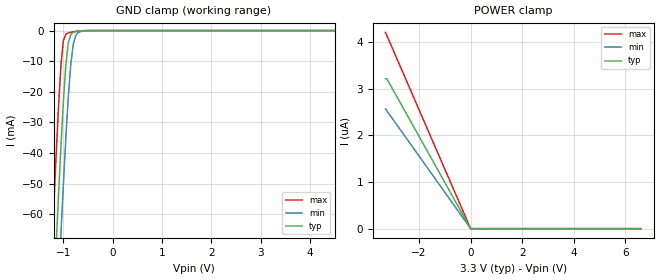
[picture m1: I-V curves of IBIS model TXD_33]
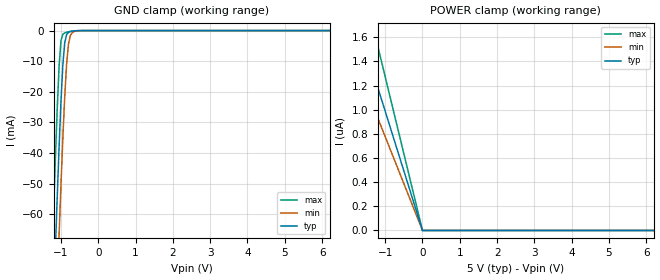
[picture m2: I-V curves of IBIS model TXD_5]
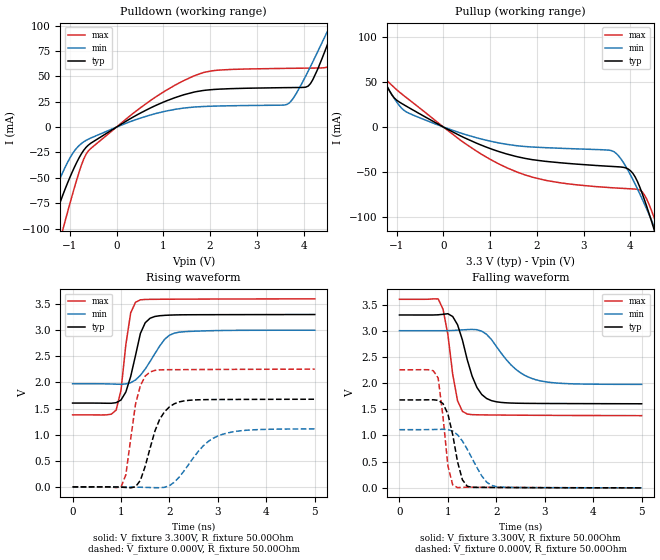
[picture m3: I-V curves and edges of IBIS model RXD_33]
| Texas Instruments Incorporated
| Isolated Dual channel Buffer
| Marketing part#   Voltage Range   Package-type   #pins/pkg drawing
| ISO7421D   3V - 5.5V   SOIC   8-pin D
| ISO7421DW   3V - 5.5V   SOIC   16-pin DW
[IBIS Ver]   4.0
[File name]   iso7421.ibs
[File Rev]   1.1
[Date]   03/17/2011
[Source]   Model built from TISPICED simulations at:
   Texas Instruments Incorporated.
   Analog-eLab, HPA
   12500 TI Blvd
   Dallas, TX -75243
   For Support e-mail: elab_ibis@list.ti.com
[Notes]   Revision History
   Rev 1.0: 11/29/2010
   - Initial model not matched to silicon
   - C_comp although listed in numberical order of value are obtained from varying PVT conditions.
   For PVT conditions for eachspecific value, refer to the buffer description under repective [Model].
   IBIS model user is responsible for using appropriate C_comp to simulate for Signal Integrity.
   Rev 1.1: 03/17/2011
   Correct signal names
   Add DW package and component
[Disclaimer] This model is designed as an aid for customers of Texas Instruments.
 TI and its licensors and suppliers make no warranties, either expressed
 or implied, with respect to this  model, including the warranties of
 merchantability or fitness for a particular purpose.
 The model is provided solely on an "as is" basis. The entire risk as to
 its quality and performance is with the customer.
[Copyright] (C)Copyright 2010 Texas Instruments Incorporated.
   All rights reserved.
|   Component ISO7421
[Component]   ISO7421D
[Manufacturer]  Texas Instruments Incorporated
[Package]   |8-pin SOIC D package
|   typ   min   max
R_pkg   0.115425   0.06126   0.16959
L_pkg   3.423325nH   2.82589nH   4.02076nH
C_pkg   0.799005pF   0.76897pF   0.82904pF
[Pin] signal_name   model_name   R_pin   L_pin   C_pin
   1  VCC1   POWER   0.067   1.914nH   0.278pF
   2  OUTA   RXD   0.062   1.816nH   0.301pF
   3  INB   TXD   0.053   1.699nH   0.298pF
   4  GND1   GND   0.067   1.907nH   0.278pF
   5  GND2   GND   0.034   1.704nH   0.311pF
   6  OUTB   RXD   0.061   1.808nH   0.310pF
   7  INA   TXD   0.062   1.817nH   0.302pF
   8  VCC2   POWER   0.034   1.716nH   0.311pF
[Pin Mapping]pulldown_ref pullup_ref gnd_clamp_ref power_clamp_ref |ext_ref
1   NC   PWRBUS1  |VCC1
2   GNDBUS1   PWRBUS1   GNDBUS1   PWRBUS1
3   NC   NC   GNDBUS1   PWRBUS1
4   GNDBUS1   NC   |GND1
5   GNDBUS2   NC   |GND2
6   NC   NC   GNDBUS1   PWRBUS1
7   GNDBUS1   PWRBUS1   GNDBUS1   PWRBUS1
8   NC   PWRBUS2  |VCC2
[Component]   ISO7421CDW
[Manufacturer]  Texas Instruments Incorporated
[Package]   |16-pin SOIC DW package
|   typ   min   max
R_pkg   0.05752   0.00646   0.11150
L_pkg   2.54064nH   1.46184nH   3.88521nH
C_pkg   0.66797pF   0.53100pF   1.09127pF
[Pin] signal_name   model_name   R_pin   L_pin   C_pin
   1  GND1   GND   0.01187   2.75369n   0.77910p
   2  NC   NC   0.00695   1.64201n   0.60891p
   3  VCC1   POWER   0.05752   2.54064n   0.66085p
   4  OUTA   RXD   0.11072   3.08476n   0.62253p
   5  INB   TXD   0.09861   2.86171n   0.61276p
   6  NC   NC   0.00646   1.46241n   0.53100p
   7  GND1   GND   0.04087   2.76190n   1.03163p
   8  NC   NC   0.07453   3.88521n   1.04445p
   9  GND2   GND   0.03985   2.89286n   1.09127p
   10  NC   NC   0.06875   2.37034n   0.80451p
   11  NC   NC   0.00646   1.46184n   0.53363p
   12  OUTB   RXD   0.11150   3.10457n   0.62303p
   13  INA   TXD   0.09893   2.86999n   0.61446p
   14  VCC2   POWER   0.05989   2.61002n   0.66797p
   15  NC   NC   0.00709   1.66297n   0.59789p
   16  GND2   GND   0.01211   2.83289n   0.79218p
[Pin Mapping]pulldown_ref pullup_ref gnd_clamp_ref power_clamp_ref |ext_ref
1   GNDBUS1   NC   |GND1
2   NC   NC
3   NC   PWRBUS1  |VCC1
4   GNDBUS1   PWRBUS1   GNDBUS1   PWRBUS1
5   NC   NC   GNDBUS1   PWRBUS1
6   NC   NC
7   GNDBUS1   NC   |GND1
8   NC   NC
9   GNDBUS2   NC   |GND2
10   NC   NC
11   NC   NC
12   GNDBUS2   PWRBUS2   GNDBUS2   PWRBUS2
13   NC   NC   GNDBUS2   PWRBUS2
14   NC   PWRBUS2  |VCC2
15   NC   NC
16   GNDBUS2   NC   |GND2
[Model Selector] TXD
TXD_33   TXD Input model for 3.0V - 3.6V
TXD_5   TXD Input model for 4.5V - 5.5V
[Model Selector] RXD
RXD_33   RXD Output model for 3.0V - 3.6V
RXD_5   RXD Output model for 4.5V - 5.5V
| Models and submodels in the file (4): TXD_33 (Input), TXD_5 (Input), RXD_33 (Output), RXD_5 (Output)
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|   TXD_33 Model
[Model]   TXD_33
Model_type   Input
|Signals   RXD
Vinh = 2.0
Vinl = 0.8
|   typ   min   max
|   (nom PVT)   (slow PVT)   (fast PVT)
C_comp   0.6217pF   0.5756pF   0.6712pF
|   typ   min   max
[Voltage Range]   3.3V   3.0V   3.6V
[Temperature Range]   27.0   136.0   -40.0
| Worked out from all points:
|   GND clamp passes 1 mA (typ) near -0.83 V on its own axis
[GND Clamp]
|   Voltage   I(typ)   I(min)   I(max)
-3.3V     -896mA     -941.7mA   -892.3mA
-1.25V    -107.4mA   -137.4mA   -77.4mA
-1.2V     -89.12mA   -119.2mA   -59.18mA
-1.15V    -71.29mA   -101.2mA   -41.62mA
-1.1V     -54.06mA   -83.57mA   -25.26mA
-1.05V    -37.76mA   -66.5mA    -11.46mA
-1V       -23.03mA   -50.19mA   -3.269mA
-950mV    -11.14mA   -35mA      -1.197mA
-900mV    -3.932mA   -21.61mA   -785uA
-800mV    -612.2uA   -4.508mA   -387.7uA
-600mV    -46.68uA   -168.3uA   -47.31uA
6.6V      0A         0A         0A
[POWER Clamp]
|   Voltage   I(typ)   I(min)   I(max)
-3.3V     3.211uA    2.564uA    4.201uA
-3.25V    3.211uA    2.525uA    4.138uA
0V        0A         0A         0A
6.6V      0A         0A         0A
|   TXD_5 Model
[Model]   TXD_5
Model_type   Input
|Signals   TXD
Vinh = 2.0
Vinl = 0.8
|   typ   min   max
|   (nom PVT)   (slow PVT)   (fast PVT)
C_comp   0.5878pF   0.5481pF   0.6309pF
|   typ   min   max
[Voltage Range]   5.0V   4.5V   5.5V
[Temperature Range]   27.0   136.0   -40.0
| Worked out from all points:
|   GND clamp passes 1 mA (typ) near -0.83 V on its own axis
[GND Clamp]
|   Voltage   I(typ)   I(min)   I(max)
-5V       -1.6A      -1.623A    -1.559A
-1.25V    -107.4mA   -137.4mA   -77.4mA
-1.2V     -89.12mA   -119.2mA   -59.18mA
-1.15V    -71.29mA   -101.2mA   -41.62mA
-1.1V     -54.06mA   -83.57mA   -25.26mA
-1.05V    -37.76mA   -66.5mA    -11.46mA
-1V       -23.04mA   -50.19mA   -3.27mA
-950mV    -11.15mA   -35mA      -1.198mA
-850mV    -1.31mA    -11.07mA   -557.5uA
-750mV    -352.2uA   -1.64mA    -261.2uA
-550mV    -20.4uA    -82.68uA   -21.52uA
10V       0A         0A         0A
[POWER Clamp]
|   Voltage   I(typ)   I(min)   I(max)
-5V       4.941uA    3.885uA    6.302uA
-2.15V    2.125uA    1.671uA    2.737uA
-2.1V     2.075uA    1.632uA    2.674uA
-1.7V     1.68uA     1.321uA    2.164uA
-1.65V    1.63uA     1.282uA    2.101uA
-1.3V     1.285uA    1.01uA     1.655uA
0V        0A         0A         0A
10V       0A         0A         0A
|   RXD_33 MODEL
[Model]   RXD_33
Model_type   Output
| Signals   RXD
Vmeas = 1.55V   |Reference voltage for timing measurements
Cref = 15pF   |Timing specification test load capacitance value
| variable   typ   min   max
|   (nom PVT)   (slow PVT)   (fast PVT)
|C_comp Average
C_comp   2.5852pF   2.2483pF   3.0761pF
|C_comp Output Low
|C_comp   2.6504pF   2.3554pF   3.1260pF
|C_comp Output High
|C_comp   2.5200pF   2.1412pF   3.0261pF
|   typ   min   max
[Voltage Range]   3.3V   3.0V   3.6V
[Temperature Range]   27.0   136.0   -40.0
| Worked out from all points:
|   slope of the pulldown table from 0 to 0.495 V, typ, clamps not added: 36.9 ohm
|   slope of the pullup table from 0 to 0.495 V, typ, clamps not added: 38.1 ohm
|   falling waveform, V_fixture 3.300V, R_fixture 50.00Ohm: 20-80 % time 334ps typ, 600ps min, 215ps max; typ from 3.3 V to 1.6 V
|   rising waveform, V_fixture 3.300V, R_fixture 50.00Ohm: 20-80 % time 269ps typ, 440ps min, 178ps max; typ from 1.6 V to 3.3 V
|   rising waveform, V_fixture 0.000V, R_fixture 50.00Ohm: 20-80 % time 354ps typ, 601ps min, 230ps max; typ from 0 V to 1.68 V
|   falling waveform, V_fixture 0.000V, R_fixture 50.00Ohm: 20-80 % time 229ps typ, 400ps min, 158ps max; typ from 1.68 V to 0 V
[Pulldown]
|   Voltage   I(typ)   I(min)   I(max)
-3.3V     -444mA     -323.4mA   -559.5mA
-1.65V    -147.4mA   -102.5mA   -196.8mA
-1.35V    -95.7mA    -66.33mA   -136mA
-1.15V    -67.06mA   -44.62mA   -101.2mA
-600mV    -17.67mA   -11.86mA   -23.39mA
1.65V     34.39mA    19.71mA    50.29mA
3.65V     38.89mA    22.42mA    57.89mA
4.15V     42.92mA    59.74mA    58.14mA
4.55V     85.96mA    98.03mA    60.72mA
4.65V     98.18mA    107.5mA    71.46mA
4.85V     122.5mA    126mA      101.8mA
6.6V      280.4mA    243.7mA    322.1mA
[Pullup]
|   Voltage   I(typ)   I(min)   I(max)
-3.3V     239.5mA    206.9mA    282.1mA
-1.95V    129.9mA    113.6mA    151.3mA
-1.7V     102.1mA    91.19mA    115.7mA
-1.3V     55.75mA    53.78mA    58.94mA
-1V       29.98mA    27.94mA    41.63mA
0V        124.8pA    622.4pA    79.46pA
1.35V     -29.93mA   -19.18mA   -45.19mA
3.65V     -44.04mA   -27.51mA   -67.78mA
4.05V     -51.38mA   -58.2mA    -68.97mA
4.3V      -80.92mA   -85.71mA   -75.5mA
4.55V     -121.4mA   -116mA     -107.4mA
6.6V      -493.8mA   -392mA     -570.7mA
[Ramp]
R_load = 50.00Ohm
|   typ   min   max
dV/dt_r   1.007V/353.701ps 666.318mV/600.696ps   1.353V/229.593ps
dV/dt_f   1.017V/334.234ps 614.806mV/599.733ps   1.333V/215.151ps
[Falling Waveform]
V_fixture = 3.300V
V_fixture_min = 3.000V
V_fixture_max = 3.600V
R_fixture = 50.00Ohm
|   Time   V(typ)   V(min)   V(max)
0s        3.3V       3V         3.6V
800ps     3.304V     3V         3.606V
900ps     3.313V     3V         3.41V
1ns       3.324V     3.001V     2.928V
1.2ns     3.113V     3.01V      1.661V
1.4ns     2.445V     3.021V     1.408V
1.6ns     1.915V     3.019V     1.395V
1.9ns     1.665V     2.831V     1.391V
2.8ns     1.612V     2.068V     1.385V
5ns       1.605V     1.975V     1.379V
[Rising Waveform]
V_fixture = 3.300V
V_fixture_min = 3.000V
V_fixture_max = 3.600V
R_fixture = 50.00Ohm
|   Time   V(typ)   V(min)   V(max)
0s        1.605V     1.975V     1.379V
900ps     1.613V     1.967V     1.471V
1ns       1.664V     1.965V     1.851V
1.1ns     1.817V     1.971V     2.723V
1.2ns     2.114V     1.995V     3.333V
1.4ns     2.937V     2.136V     3.582V
1.6ns     3.229V     2.4V       3.591V
1.9ns     3.284V     2.825V     3.593V
2.1ns     3.292V     2.943V     3.594V
5ns       3.3V       3V         3.6V
[Rising Waveform]
V_fixture = 0.000V
V_fixture_min = 0.000V
V_fixture_max = 0.000V
R_fixture = 50.00Ohm
|   Time   V(typ)   V(min)   V(max)
0s        336.7pV    705.2pV    374.2pV
1ns       -5.097mV   157.2uV    -2.804mV
1.1ns     -10.77mV   -533.8uV   231mV
1.3ns     2.172mV    -3.954mV   1.586V
1.4ns     125.6mV    -6.338mV   1.939V
1.6ns     740.1mV    -11.61mV   2.201V
1.8ns     1.298V     -16.07mV   2.24V
2.2ns     1.626V     186mV      2.245V
3ns       1.673V     975.1mV    2.249V
5ns       1.678V     1.111V     2.254V
[Falling Waveform]
V_fixture = 0.000V
V_fixture_min = 0.000V
V_fixture_max = 0.000V
R_fixture = 50.00Ohm
|   Time   V(typ)   V(min)   V(max)
0s        1.678V     1.111V     2.254V
700ps     1.681V     1.113V     2.235V
800ps     1.67V      1.116V     2.097V
1ns       1.412V     1.112V     422.2mV
1.1ns     1.014V     1.084V     56.58mV
1.2ns     495.5mV    1.013V     4.556mV
1.3ns     153.7mV    894mV      9.242mV
1.4ns     30.49mV    736.9mV    12.55mV
1.9ns     7.265mV    47.26mV    9.425mV
5ns       336.7pV    705.2pV    374.2pV
